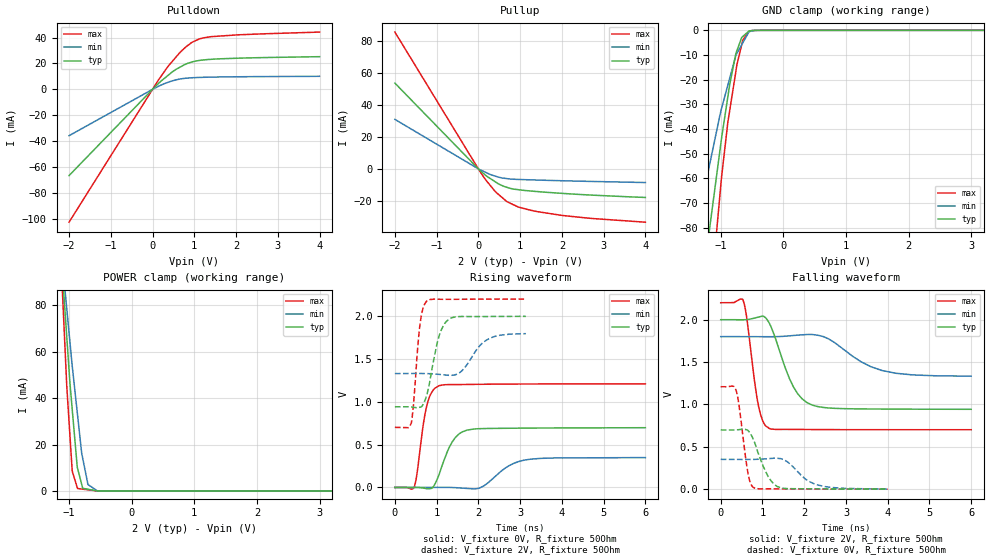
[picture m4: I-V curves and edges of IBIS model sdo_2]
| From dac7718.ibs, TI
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|   sdo_2 Model
[Model]   sdo_2
Model_type   3-state
Polarity   Non-Inverting
Vmeas = 1.0
Vref = 1.0
Cref = 5pF
Rref = 50
|   typ   min   max
|   (Nom PVT)   (Fast PVT)   (Slow PVT)
|C_comp from frequency method(F=50MHz)
|Average
C_comp   4.066e-12   3.022e-12   4.946e-12
|ON state : BUFFER OUTPUT TURNED HIGH
|C_comp   4.386e-12   3.359e-12   5.296e-12
|OFF state: BUFFER IN HIGH IMPEDANCE
|C_comp   4.066e-12   3.022e-12   4.946e-12
|C_comp from LC Tank Method (L=1nH)
|Resonant Frequency(Hz)   2.75e9   3.13e9   2.49e9
|C_comp   3.353e-12   2.588e-12   4.090e-12
| Where nom  PVT is Nominal Process,  2V,  33C
|   Fast PVT is Strong Process,   2.2V,  -40C
|   Slow PVT is Weak Process,   1.8V,  113C
[Voltage Range]   2   1.8   2.2
|Ambient Temperature   25   85   -40
|Junction Temperature
[Temperature Range]   33   113   -40
[Pullup Reference]   2   1.8   2.2
[Pulldown Reference]   0   0   0
[Power Clamp Reference]   2   1.8   2.2
[GND Clamp Reference]   0   0   0
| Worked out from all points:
|   slope of the pulldown table from 0 to 0.3 V, typ, clamps not added: 33.6 ohm
|   slope of the pullup table from 0 to 0.3 V, typ, clamps not added: 47.6 ohm
|   GND clamp passes 1 mA (typ) near -0.58 V on its own axis
|   POWER clamp passes 1 mA (typ) near -0.75 V on its own axis
|   falling waveform, V_fixture 2V, R_fixture 50Ohm: 20-80 % time 504ps typ, 915ps min, 242ps max; typ from 2 V to 0.943 V
|   rising waveform, V_fixture 0V, R_fixture 50Ohm: 20-80 % time 362ps typ, 569ps min, 219ps max; typ from 0 V to 0.698 V
|   rising waveform, V_fixture 2V, R_fixture 50Ohm: 20-80 % time 270ps typ, 433ps min, 150ps max; typ from 0.942 V to 2 V
|   falling waveform, V_fixture 0V, R_fixture 50Ohm: 20-80 % time 344ps typ, 507ps min, 190ps max; typ from 0.699 V to 0 V
[Pulldown]
|   Voltage   I(typ)   I(min)   I(max)
-2V       -66.72mA   -35.85mA   -102.8mA
149.6mV   4.771mA    2.435mA    7.622mA
387.2mV   11.22mA    5.629mA    18.43mA
655.6mV   17.14mA    7.974mA    28.5mA
930.6mV   21.04mA    8.938mA    36.07mA
1.122V    22.35mA    9.209mA    39.02mA
1.419V    23.25mA    9.452mA    40.78mA
2.077V    24.11mA    9.731mA    42.2mA
4V        25.26mA    10.08mA    44.28mA
[GND Clamp]
|   Voltage   I(typ)   I(min)   I(max)
-2V       -261.5mA   -168.2mA   -375.4mA
-1.375V   -121.6mA   -79.19mA   -175.9mA
-1.172V   -79.27mA   -53.77mA   -112.9mA
-1.115V   -68.41mA   -46.89mA   -95.58mA
-1.015V   -49.17mA   -34.71mA   -67.43mA
-985.6mV  -43.54mA   -31.53mA   -59.22mA
-886.6mV  -26.99mA   -22.24mA   -37.35mA
-856mV    -21.89mA   -19.37mA   -32.42mA
-758mV    -9.445mA   -10.18mA   -16.64mA
-646.8mV  -2.474mA   -5.038mA   -3.962mA
-550mV    -301uA     -688.1uA   -431.3uA
4V        0A         0A         0A
[Pullup]
|   Voltage   I(typ)   I(min)   I(max)
-2V       53.75mA    31.02mA    85.71mA
105.6mV   -2.547mA   -1.353mA   -4.277mA
387.2mV   -7.792mA   -4.404mA   -13.68mA
482mV     -9.409mA   -5.186mA   -16.03mA
668.8mV   -11.44mA   -6.045mA   -20.18mA
950.4mV   -13.02mA   -6.607mA   -23.84mA
1.232V    -13.81mA   -6.848mA   -25.81mA
1.976V    -15.28mA   -7.409mA   -29.05mA
2.752V    -16.48mA   -7.892mA   -31.14mA
4V        -17.91mA   -8.557mA   -33.4mA
[POWER Clamp]
|   Voltage   I(typ)   I(min)   I(max)
-2V       307.1mA    278.7mA    353.9mA
-1.327V   180.8mA    160.7mA    214.8mA
-1.036V   66.3mA     78.4mA     45.05mA
-986mV    46.5mA     64.18mA    23.93mA
-950.4mV  35.47mA    54.1mA     8.954mA
-870mV    10.55mA    34.1mA     1.513mA
-864.6mV  9.78mA     32.76mA    1.035mA
-797.4mV  2.748mA    16.13mA    813.7uA
-782mV    1.137mA    14.05mA    763.1uA
-698.4mV  727.4uA    2.769mA    488.1uA
-549mV    808.5nA    43.33uA    67.74nA
4V        0A         0A         0A
[Ramp]
R_load = 50
|   typ   min   max
dV/dt_r   0.418516/3.59034e-10   0.209195/5.6627e-10   0.725423/2.18501e-10
dV/dt_f   0.634424/5.00726e-10   0.279952/8.99491e-10   0.899108/2.41964e-10
[Falling Waveform]
V_fixture = 2V
V_fixture_min = 1.8V
V_fixture_max = 2.2V
R_fixture = 50Ohm
|   Time   V(typ)   V(min)   V(max)
0s        2V         1.8V       2.2V
538ps     1.999V     1.8V       2.227V
622ps     2.001V     1.8V       2.026V
904ps     2.031V     1.8V       984.4mV
1.026ns   2.04V      1.799V     785.5mV
1.164ns   1.959V     1.799V     716.6mV
1.742ns   1.207V     1.814V     705.3mV
2.174ns   996.3mV    1.826V     703.9mV
3.868ns   945.4mV    1.4V       701.8mV
6ns       942.6mV    1.333V     701.5mV
[Rising Waveform]
V_fixture = 0V
V_fixture_min = 0V
V_fixture_max = 0V
R_fixture = 50Ohm
|   Time   V(typ)   V(min)   V(max)
0s        1.047nV    1.522nV    844.5pV
458ps     851.1uV    -15.42uV   -3.768mV
762ps     -14.94mV   275.5uV    949.4mV
898ps     -4.721mV   453.7uV    1.123V
1.052ns   143mV      621.8uV    1.187V
1.376ns   534mV      -770.6uV   1.201V
1.73ns    669.8mV    -11.82mV   1.202V
2.034ns   686.4mV    -5.835mV   1.204V
3.1ns     692.6mV    318.8mV    1.208V
6ns       697.5mV    348.7mV    1.209V
[Rising Waveform]
V_fixture = 2V
V_fixture_min = 1.8V
V_fixture_max = 2.2V
R_fixture = 50Ohm
|   Time   V(typ)   V(min)   V(max)
0s        941.6mV    1.33V      701.5mV
392ps     939.2mV    1.33V      748.8mV
590ps     935.9mV    1.331V     1.857V
668ps     963.4mV    1.33V      2.081V
764ps     1.078V     1.329V     2.176V
1.066ns   1.78V      1.32V      2.198V
1.282ns   1.96V      1.31V      2.196V
1.592ns   1.996V     1.356V     2.197V
2.272ns   1.996V     1.741V     2.199V
3.136ns   1.998V     1.796V     2.2V
[Falling Waveform]
V_fixture = 0V
V_fixture_min = 0V
V_fixture_max = 0V
R_fixture = 50Ohm
|   Time   V(typ)   V(min)   V(max)
0s        698.7mV    351.4mV    1.209V
308ps     698.1mV    351mV      1.213V
372ps     699.4mV    350.9mV    1.159V
434ps     702.3mV    350.8mV    1.006V
656ps     690.9mV    350.7mV    177.8mV
780ps     589.4mV    351.4mV    21.9mV
1.136ns   150.3mV    359.8mV    4.305mV
1.434ns   16.41mV    360.2mV    3.293mV
2.334ns   3.428mV    47.78mV    1.23mV
4ns       482.5uV    1.282mV    26.66uV
